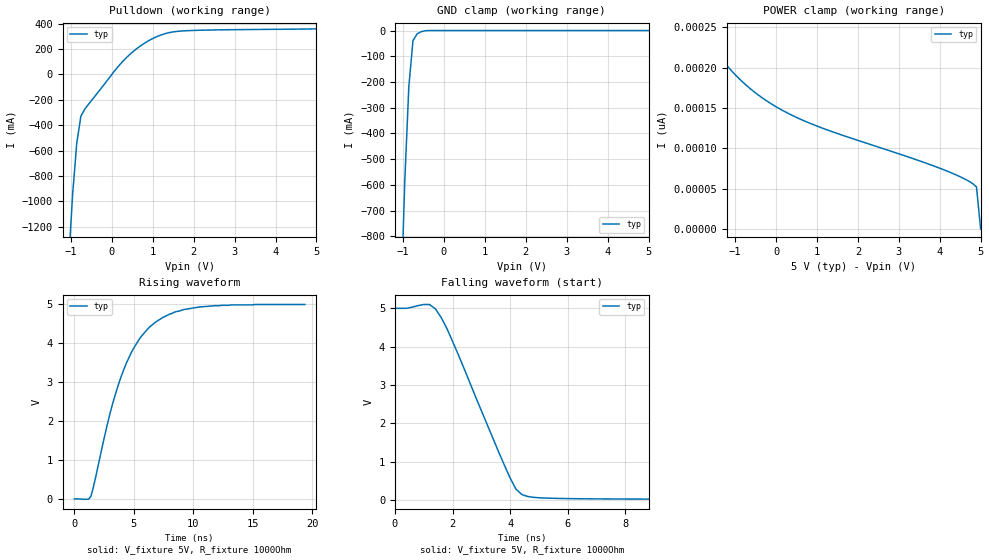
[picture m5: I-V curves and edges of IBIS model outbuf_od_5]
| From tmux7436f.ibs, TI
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| outbuf_od_5
[Model]   outbuf_od_5
Model_type   Open_drain
Polarity   Inverting
Vmeas = 2.5
Vref = 5
Cref = 2pF
Rref = 1000
|   typ   min   max
C_comp   2.533030e-12   NA   NA
| Where nom  PVT is Nominal Process, 5.0, 27C
[Voltage Range]   5   NA   NA
[Temperature Range]   27   NA   NA
[Pullup Reference]   5   NA   NA
[Pulldown Reference]   0   NA   NA
[Power Clamp Reference]   5   NA   NA
[GND Clamp Reference]   0   NA   NA
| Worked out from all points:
|   slope of the pulldown table from 0 to 0.75 V, typ, clamps not added: 3.18 ohm
|   GND clamp passes 1 mA (typ) near -0.46 V on its own axis
|   falling waveform, V_fixture 5V, R_fixture 1000Ohm: 20-80 % time 1.66ns typ, NA min, NA max; typ from 5 V to 0.012 V
|   rising waveform, V_fixture 5V, R_fixture 1000Ohm: 20-80 % time 3.14ns typ, NA min, NA max; typ from 0.012 V to 5 V
[Pulldown]
|   Voltage   I(typ)   I(min)   I(max)
-5V       -29.62A    NA         NA
-1.061V   -1.498A    NA         NA
-959.6mV  -946.7mA   NA         NA
-858.6mV  -541.8mA   NA         NA
-757.6mV  -329.1mA   NA         NA
-656.6mV  -270.7mA   NA         NA
50.51mV   21.22mA    NA         NA
252.5mV   97.64mA    NA         NA
555.6mV   189.5mA    NA         NA
1.061V    291.9mA    NA         NA
1.566V    337.6mA    NA         NA
5V        358.7mA    NA         NA
[GND Clamp]
|   Voltage   I(typ)   I(min)   I(max)
-5V       -28.73A    NA         NA
-1.061V   -1.118A    NA         NA
-959.6mV  -593.3mA   NA         NA
-858.6mV  -218.3mA   NA         NA
-757.6mV  -39.58mA   NA         NA
-656.6mV  -12.91mA   NA         NA
-555.6mV  -4.466mA   NA         NA
-353.5mV  -46.56uA   NA         NA
5V        151.6pA    NA         NA
[POWER Clamp]
|   Voltage   I(typ)   I(min)   I(max)
-5V       6.654nA    NA         NA
-1.768V   245.7pA    NA         NA
-1.364V   213.2pA    NA         NA
-959.6mV  189.3pA    NA         NA
-454.6mV  166.9pA    NA         NA
50.51mV   150.1pA    NA         NA
959.6mV   128.4pA    NA         NA
3.788V    79.38pA    NA         NA
4.394V    67.2pA     NA         NA
4.798V    56.62pA    NA         NA
4.899V    52.12pA    NA         NA
5V        0A         NA         NA
[Ramp]
R_load = 1000
|   typ   min   max
dV/dt_r   2.94/3.2e-9   NA   NA
dV/dt_f   2.89/1.6e-09   NA   NA
[Falling Waveform]
V_fixture = 5V
V_fixture_min = 5V
V_fixture_max = 5V
R_fixture = 1000Ohm
C_fixture = 0F
Time		V(typ)		V(min)		V(max)
0s        5V         NA         NA
1.2ns     5.1V       NA         NA
1.4ns     4.99V      NA         NA
1.6ns     4.77V      NA         NA
2ns       4.14V      NA         NA
4ns       568mV      NA         NA
4.2ns     279mV      NA         NA
4.6ns     87.5mV     NA         NA
7ns       24mV       NA         NA
19.6ns    12.4mV     NA         NA
[Rising Waveform]
V_fixture = 5V
V_fixture_min = 5VV
V_fixture_max = 5V
R_fixture = 1000Ohm
C_fixture = 0F
Time		V(typ)		V(min)		V(max)
0s        11.7mV     NA         NA
1.2ns     6.34mV     NA         NA
1.4ns     81mV       NA         NA
3ns       2.2V       NA         NA
3.8ns     3.03V      NA         NA
5ns       3.88V      NA         NA
6.4ns     4.44V      NA         NA
8.4ns     4.8V       NA         NA
10.6ns    4.94V      NA         NA
19.4ns    5V         NA         NA
